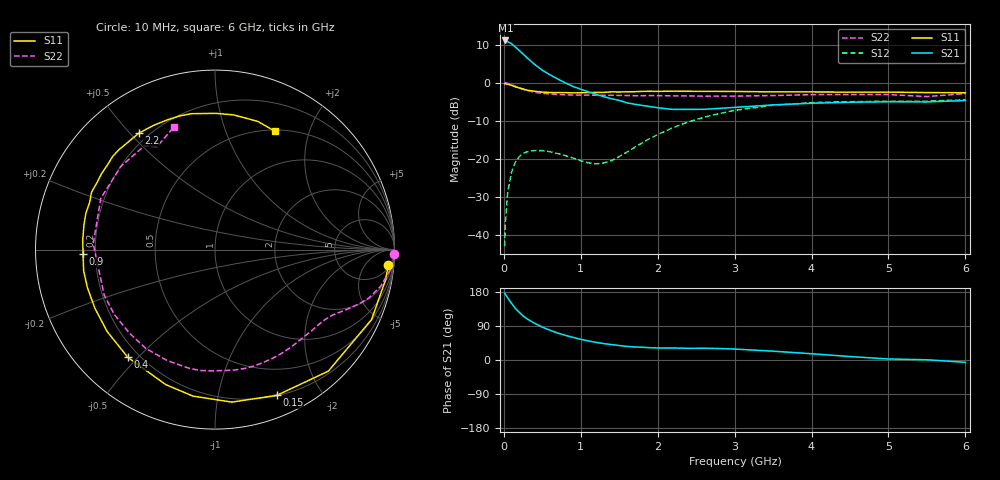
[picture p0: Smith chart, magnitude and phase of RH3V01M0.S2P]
! SIEMENS Small Signal Semiconductors
! BFR106
! Si NPN RF Bipolar Junction Transistor in SOT23
! VCE = 3 V  IC = 1 mA
! Common Emitter S-Parameters:  August  1996
# GHz  S  MA  R  50
!  f  S11  S21  S12  S22
! GHz  MAG  ANG  MAG  ANG  MAG  ANG  MAG  ANG
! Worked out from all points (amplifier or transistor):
!   36 points, 10 MHz to 6 GHz, reference 50 ohm
!   highest |S21| = 11.1 dB at 20 MHz (marker M1)
!   |S21| within 3 dB of that: start of sweep to 220.6 MHz
!   unconditionally stable (mu >= 1): 858.8 MHz to end of sweep
!   at 250 MHz: K = 0.26, MSG = 13.0 dB, |S12| = -18.6 dB
!   at 1.4 GHz: K = 1.44, MAG = 4.2 dB, |S12| = -20.4 dB
!   at 6 GHz: K = 1.02, MAG = -0.9 dB, |S12| = -4.5 dB
!   S11 on the Smith chart (normalised r, x): 10 MHz: 7, -20; 150 MHz: 0.20, -1.49; 400 MHz: 0.16, -0.47; 900 MHz: 0.15, -0.02; 2.2 GHz: 0.16, +0.53; 6 GHz: 0.52, +1.50
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0.01  0.9685 -5.0  3.574 176.2  0.0072 89.0  0.999 -1.5
0.02  0.9659 -9.8  3.582 173.7  0.0147 83.2  0.9995 -2.8
0.05  0.9556 -24.0  3.46 163.7  0.0365 75.6  0.9821 -6.7
0.1  0.9259 -47.0  3.245 149.8  0.0675 64.1  0.9451 -12.5
0.15  0.882 -67.0  2.942 136.1  0.0914 52.5  0.9003 -17.3
0.2  0.8549 -83.7  2.651 126.0  0.1073 44.3  0.8598 -20.5
0.25  0.8254 -98.6  2.38 116.2  0.1181 37.1  0.8199 -23.4
0.3  0.8006 -110.1  2.127 109.0  0.1242 32.2  0.7919 -25.5
0.4  0.7722 -129.0  1.742 96.9  0.1295 23.9  0.75 -29.1
0.5  0.7546 -142.8  1.459 86.7  0.1287 18.5  0.726 -32.5
0.6  0.7446 -154.1  1.271 78.5  0.1247 15.5  0.7116 -36.2
0.9  0.7355 -178.0  0.894 59.7  0.1029 16.4  0.6904 -48.1
1.1  0.7428 169.6  0.76 50.2  0.089 26.7  0.687 -57.2
1.3  0.7464 159.3  0.656 43.2  0.0888 45.0  0.6836 -66.4
1.6  0.7608 146.1  0.545 35.9  0.1234 66.8  0.6796 -81.2
2.2  0.7752 123.3  0.447 31.6  0.2582 69.4  0.6732 -113.3
2.8  0.7704 104.6  0.461 30.3  0.3943 55.1  0.6675 -147.3
3.5  0.7591 89.7  0.512 23.3  0.5075 36.6  0.679 177.3
4.5  0.7521 76.4  0.555 9.1  0.5648 14.6  0.6998 138.4
5  0.7528 71.5  0.563 2.7  0.5715 6.7  0.6993 124.4
5.5  0.7428 66.5  0.56 0.6  0.5743 3.0  0.6586 119.4
6  0.7391 63.1  0.584 -6.2  0.5971 -4.8  0.7197 108.6
